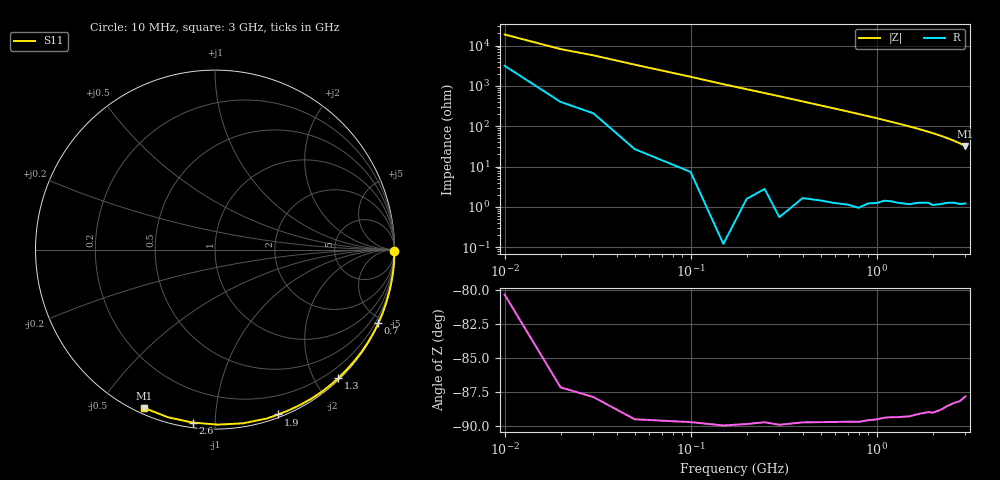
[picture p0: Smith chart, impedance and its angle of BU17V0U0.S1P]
! SIEMENS Small Signal Semiconductors
! BB833
! Si Tuning Diode in SOD323
! VR = 17 V
! S-Parameters:  April  1996
# GHz  S  MA  R  50
!  f  S11
! GHz  MAG  ANG
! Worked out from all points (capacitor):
!   31 points, 10 MHz to 3 GHz, reference 50 ohm
!   read as one part to ground: C = 927 fF near 10 MHz
!   lowest |Z| = 32.5 ohm at 3 GHz (marker M1)
!   S11 on the Smith chart (normalised r, x): 10 MHz: open; 700 MHz: 0.02, -4.64; 1.3 GHz: 0.03, -2.35; 1.9 GHz: 0.03, -1.45; 2.6 GHz: 0.03, -0.88; 3 GHz: 0.02, -0.65
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0.01  0.9991 -0.3
0.02  0.9994 -0.7
0.1  0.9997 -3.4
0.15  1 -5.2
0.2  0.9998 -6.9
0.3  0.9998 -10.3
0.4  0.999 -13.8
0.5  0.9987 -17.3
0.6  0.9984 -20.8
0.7  0.998 -24.3
0.8  0.9978 -27.9
0.9  0.9964 -31.4
1  0.9955 -35.0
1.1  0.9937 -38.7
1.2  0.9928 -42.4
1.3  0.9922 -46.1
1.4  0.9914 -49.8
1.5  0.9906 -53.5
1.6  0.9887 -57.3
1.7  0.9868 -61.1
1.8  0.9854 -65.1
1.9  0.9839 -69.0
2  0.9843 -72.9
2.2  0.9804 -80.9
2.4  0.9752 -89.1
2.6  0.9717 -97.4
2.8  0.9702 -105.7
3  0.9663 -114.0
